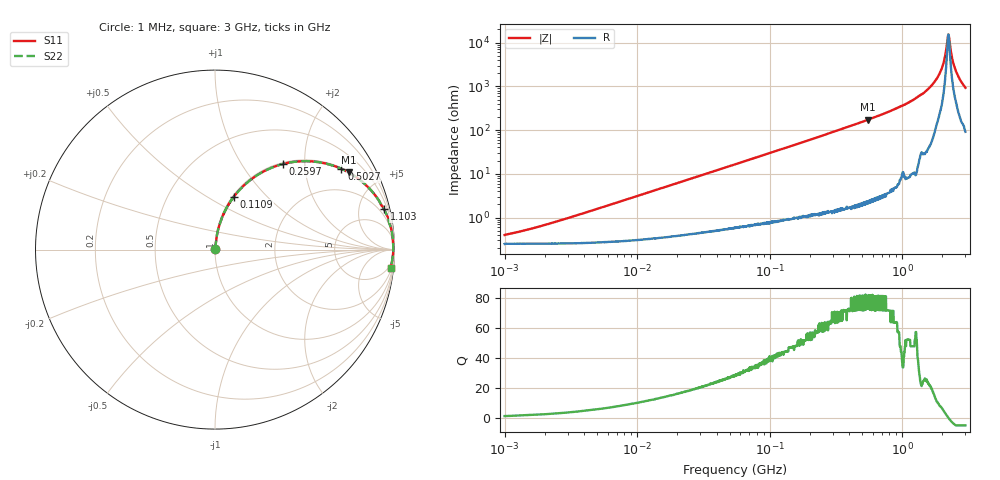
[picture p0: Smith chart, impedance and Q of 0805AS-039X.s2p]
!s-Parameter Generated by FASTRON Sdn. Bhd.
!FASTRON P/N : 0805AS-039X
!Keysight Technologies: E4991B_MY54100416_A.01.15
!Date: Mon Jun 15 12:50:25 2026
!Version  :Rev01  Mon Jun 15 12:50:25 2026
!Data & Calibration Information:
!Freq  S11  S21  S12  S22
!PortZ  Port1:50+j0  Port2:50+j0
!When reading reference impedance value at option line is always used.
! Remarks : This data is being provided solely for informational purposes.
# Hz S dB R 50
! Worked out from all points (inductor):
!   1601 points, 1 MHz to 3 GHz, reference 50 ohm
!   read as one part in series: L = 49.7 nH near 2.449 MHz
!   highest Q = 81.4 at 552.8 MHz (marker M1), where L = 49.6 nH
!   self-resonance near 2.233 GHz
!   S11 on the Smith chart (normalised r, x): 1 MHz: 1.00, +0.01; 110.9 MHz: 1.02, +0.66; 259.7 MHz: 1.03, +1.55; 502.7 MHz: 1.04, +3.10; 1.103 GHz: 1.15, +8.36; 3 GHz: 3, -19
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1000000  -48.00 51.2  -0.02 -0.2  -0.02 -0.2  -48.00 51.2
3804036  -38.30 76.9  -0.02 -0.7  -0.02 -0.7  -38.30 76.9
1.447069e7  -27.10 83.1  -0.04 -2.5  -0.04 -2.5  -27.10 83.1
5.504702e7  -15.80 78.7  -0.17 -9.3  -0.17 -9.3  -15.80 78.7
1.109129e8  -10.10 70.4  -0.51 -18.2  -0.51 -18.2  -10.10 70.4
2.083556e8  -5.63 57.4  -1.49 -31.5  -1.49 -31.5  -5.63 57.4
2.596726e8  -4.32 51.6  -2.11 -37.5  -2.11 -37.5  -4.32 51.6
5.026765e8  -1.56 32.6  -5.37 -56.7  -5.37 -56.7  -1.56 32.6
5.528145e8  -1.31 30.0  -6.03 -59.3  -6.03 -59.3  -1.31 30.0
7.925923e8  -0.62 20.7  -9.05 -68.5  -9.05 -68.5  -0.62 20.7
1.10276e9  -0.28 13.4  -12.70 -75.5  -12.70 -75.5  -0.28 13.4
1.481494e9  -0.12 7.6  -17.50 -80.2  -17.50 -80.2  -0.12 7.6
1.800756e9  -0.07 4.0  -23.20 -81.3  -23.20 -81.3  -0.07 4.0
2.000286e9  -0.06 2.1  -28.60 -79.0  -28.60 -79.0  -0.06 2.1
2.081985e9  -0.05 1.4  -32.30 -74.7  -32.30 -74.7  -0.05 1.4
2.177892e9  -0.05 0.5  -39.40 -54.0  -39.40 -54.0  -0.05 0.5
2.23307e9  -0.06 0.0  -43.80 -3.6  -43.80 -3.6  -0.06 0.0
2.289646e9  -0.06 -0.5  -39.70 49.5  -39.70 49.5  -0.06 -0.5
2.41921e9  -0.07 -1.5  -31.10 72.4  -31.10 72.4  -0.07 -1.5
2.543347e9  -0.08 -2.5  -27.10 76.2  -27.10 76.2  -0.08 -2.5
2.769173e9  -0.11 -4.2  -22.50 78.5  -22.50 78.5  -0.11 -4.2
3e9  -0.14 -6.0  -19.50 78.3  -19.50 78.3  -0.14 -6.0
